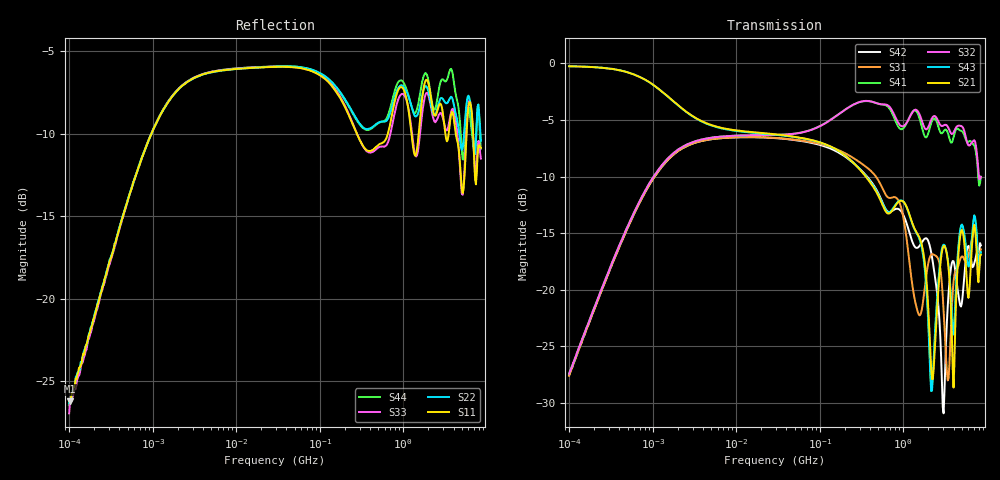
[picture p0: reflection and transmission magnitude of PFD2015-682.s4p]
# MHz S MA R 50
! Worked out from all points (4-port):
!   498 points, 100 kHz to 8.5 GHz, reference 50 ohm
!   strongest paths, dB at 100 kHz, 1.698 MHz, 29.49 MHz, 500.7 MHz, 8.5 GHz:
!     S21: -0.3, -3.2, -6.3, -11.7, -16.9
!     S43: -0.2, -3.2, -6.3, -11.6, -16.7
!     S32: -27.4, -8.1, -6.3, -3.6, -10.0
!     S41: -27.5, -8.1, -6.3, -3.6, -10.0
!     S31: -27.6, -8.2, -6.6, -10.3, -16.4
!     S42: -27.6, -8.2, -6.6, -11.4, -16.1
!   lowest |S11| = -26.2 dB at 102.3 kHz (marker M1), VSWR 1.10, Z = 52.4 + j4.43 ohm
!   |S11| at or under -10 dB: 277.5 MHz to 654.5 MHz (377 MHz wide, 80.9 % of centre); 4.249 GHz to 5.735 GHz (1.486 GHz wide, 29.8 % of centre); 6.856 GHz to end of sweep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
0.1  0.04902 59.4  0.9715 -2.5  0.04164 -95.7  0.04237 84.0
     0.9715 -2.5  0.04838 61.4  0.04249 83.6  0.04192 -96.4
     0.04164 -95.7  0.04249 83.6  0.04502 59.8  0.9723 -2.5
     0.04237 84.0  0.04192 -96.4  0.9723 -2.5  0.04769 62.0
0.1023101  0.04899 59.4  0.9713 -2.6  0.0428 -95.9  0.04351 83.8
           0.9713 -2.6  0.04958 61.9  0.04354 83.8  0.04287 -96.2
           0.0428 -95.9  0.04354 83.8  0.0486 60.1  0.9714 -2.6
           0.04351 83.8  0.04287 -96.2  0.9714 -2.6  0.04806 61.5
241.0775  0.3431 -50.9  0.3701 -103.5  0.3859 72.0  0.6513 -23.3
          0.3701 -103.5  0.3713 -45.1  0.6514 -22.7  0.3684 79.2
          0.3859 72.0  0.6514 -22.7  0.3457 -51.5  0.3704 -103.1
          0.6513 -23.3  0.3684 79.2  0.3704 -103.1  0.3684 -43.8
1399.167  0.2707 170.7  0.1829 -121.8  0.0874 85.6  0.6195 174.0
          0.1829 -121.8  0.3562 170.8  0.6245 176.9  0.1537 38.7
          0.0874 85.6  0.6245 176.9  0.2714 164.0  0.1817 -117.5
          0.6195 174.0  0.1537 38.7  0.1817 -117.5  0.3654 172.5
2652.059  0.3819 17.2  0.1042 148.4  0.1352 47.9  0.5206 10.8
          0.1042 148.4  0.3905 20.0  0.551 12.5  0.08206 37.7
          0.1352 47.9  0.551 12.5  0.359 13.0  0.1128 142.8
          0.5206 10.8  0.08206 37.7  0.1128 142.8  0.4257 10.2
4187.455  0.3242 -173.9  0.06704 -69.8  0.1202 -120.5  0.5016 -176.1
          0.06704 -69.8  0.369 -177.9  0.5125 -179.1  0.1223 -110.7
          0.1202 -120.5  0.5125 -179.1  0.3531 -179.2  0.08623 -82.8
          0.5016 -176.1  0.1223 -110.7  0.08623 -82.8  0.4241 175.9
8500  0.2864 -47.2  0.1425 58.4  0.1507 11.2  0.3156 -15.1
      0.1425 58.4  0.3005 -65.5  0.3154 -18.6  0.1569 13.5
      0.1507 11.2  0.3154 -18.6  0.2657 -71.2  0.1463 38.5
      0.3156 -15.1  0.1569 13.5  0.1463 38.5  0.2845 -61.7
